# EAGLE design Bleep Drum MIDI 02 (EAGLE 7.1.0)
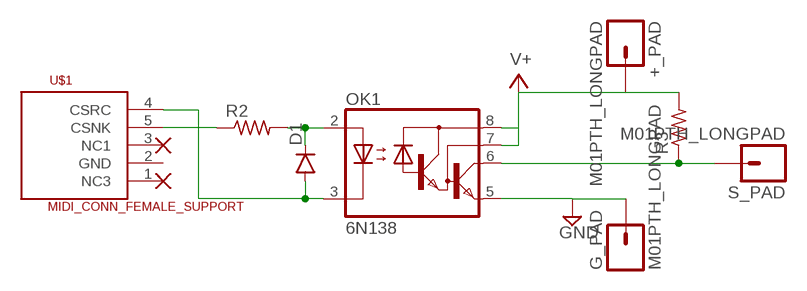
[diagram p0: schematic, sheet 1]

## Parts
+_PAD  M01PTH_LONGPAD  [1X01_LONGPAD]
D1  DIODE1N4148  [DIODE-1N4148]
G_PAD  M01PTH_LONGPAD  [1X01_LONGPAD]
OK1  6N138  [DIL08]
R2  R-US_0204/5  [0204/5]
R3  R-US_0204/5  [0204/5]
S_PAD  M01PTH_LONGPAD  [1X01_LONGPAD]
U$1  MIDI_CONN_FEMALE_SUPPORT  [DIN_5_FEMALE_SUPPORT]

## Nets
GND: G_PAD.1 OK1.5(GND)
N$1: R2.1 U$1.5(CSNK)
N$2: D1.C OK1.2(A) R2.2
N$6: OK1.6(VO) R3.1 S_PAD.1
N$8: D1.A OK1.3(C) U$1.4(CSRC)
V+: +_PAD.1 OK1.7(VB) OK1.8(VCC) R3.2
Unconnected: U$1.1(NC3) U$1.2(GND) U$1.3(NC1)

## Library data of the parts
+_PAD G_PAD S_PAD = SparkFun-Connectors:M01: Header 1
D1 = SparkFun-DiscreteSemi:DIODE: Diode
OK1 = optocoupler:6N138: MOTOROLA OPTO COUPLER; MF: VISHAY/TELEFUNKEN; MPN: 6N138; OC_FARNELL: 9860150; OC_NEWARK: 35K5294
R2 R3 = adafruit:R-US_: RESISTOR, American symbol
U$1 = SparkFun-Connectors:MIDI_CONN_FEMALE_SUPPORT: MIDI connector with strain relief (DIN-5 female)

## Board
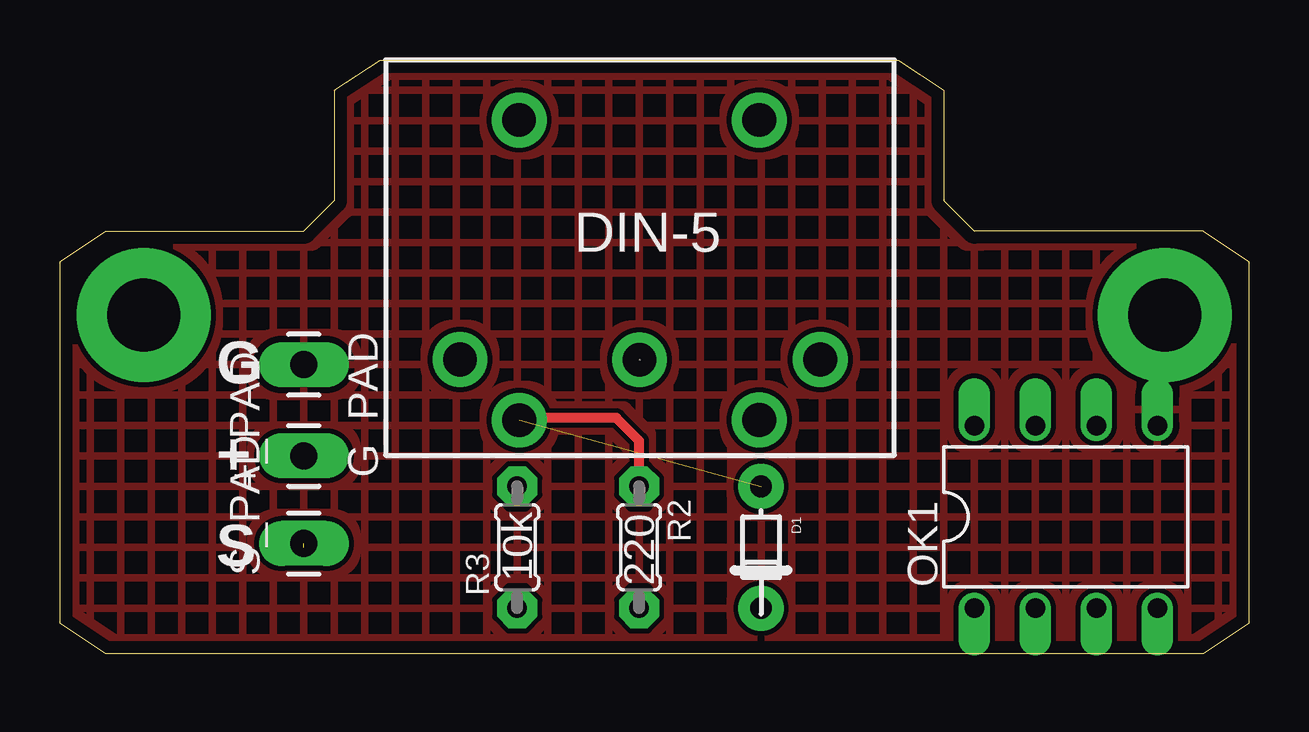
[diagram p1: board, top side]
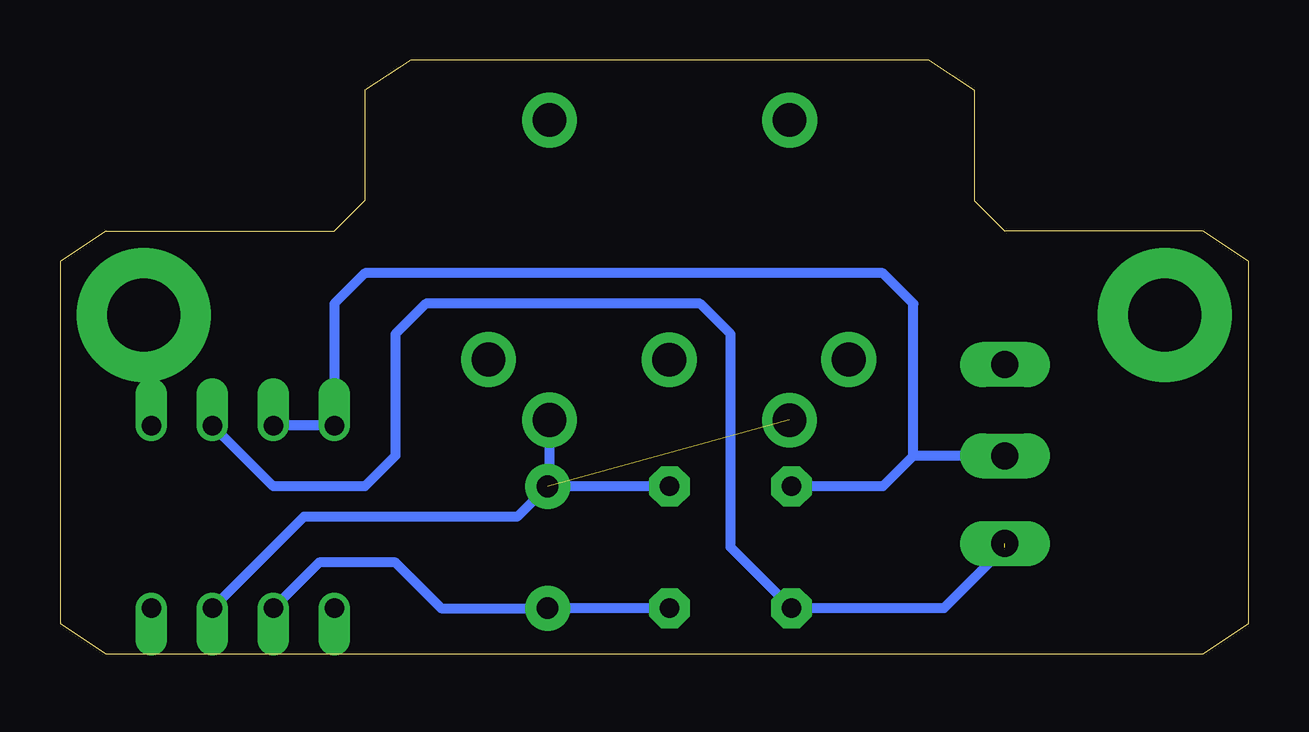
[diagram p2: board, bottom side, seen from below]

Size 49.53 x 24.77 mm. Coordinates in mm from the lower left corner, seen from the top.
Outline: 13.34,24.77 34.93,24.77 36.83,23.49 36.83,18.89 38.1,17.62 47.62,17.62 49.53,16.35 49.53,1.27 47.62,0 1.91,0 0,1.27 0,16.35 1.91,17.62 10.16,17.62 11.43,18.89 11.43,23.49 13.34,24.77
Copper layers (1*16): Top 0.035mm / dielectric 1.5mm / Bottom 0.035mm
Design rules "default": minimum track width 12mil, minimum drill 15mil, track to track 8mil, track to pad 8mil, pad to pad 8mil, via to via 8mil, smd to smd 8mil, copper to edge 20mil, drill to drill 8mil, minimum pad ring 10mil, minimum via ring 8mil, stop-mask expansion 4mil, vias tented up to drill 0mil, thermal gap 10mil

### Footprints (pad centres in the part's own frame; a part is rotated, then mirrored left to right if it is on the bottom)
1X01_LONGPAD = drill 1.118 pad 1.88 long: 1 0,0
DIODE-1N4148 = drill 0.9 pad 1.88: A -3.81,0; C 1.27,0
DIL08 = drill 0.813 offset: 1 -3.81,-3.81; 2 -1.27,-3.81; 3 1.27,-3.81; 4 3.81,-3.81; 5 3.81,3.81; 6 1.27,3.81; 7 -1.27,3.81; 8 -3.81,3.81
0204/5 = drill 0.813 pad 1.676 octagon: 1 -2.54,0; 2 2.54,0
DIN_5_FEMALE_SUPPORT = drill 1.4 pad 2.286: 1 7.94,3.6; 2 0.46,3.61; 3 -7.07,3.6; 4 5.47,6.13; 5 -4.53,6.12; 6 -4.53,-6.382; 7 5.478,-6.382

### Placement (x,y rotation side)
+_PAD  10.16,8.26 90 top
D1  29.21,3.17 270 top
G_PAD  10.16,12.07 270 top
OK1  41.91,5.71 0 top
R2  24.13,4.44 270 top
R3  19.05,4.44 90 top
S_PAD  10.16,4.6 90 top
U$1  24.61,15.88 180 top

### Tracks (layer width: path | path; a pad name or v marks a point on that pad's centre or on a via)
GND
  pour Top (hatched): -2.54,-0.64 -2.54,25.24 50.8,25.24 50.8,-1.91
N$1
  Top 0.406: R2.1 24.13,8.89 23.18,9.84 19.05,9.84
  Bottom 0.406: U$1.5 29.14,7.06 29.21,6.99 R2.1
N$2
  Bottom 0.406: OK1.2 38.73,3.81 35.56,3.81 33.66,1.91 D1.C R2.2
N$6  (1 unrouted)
  Bottom 0.406: 10.16,4.44 12.7,1.91 16.51,1.91 R3.1 | R3.1 21.59,4.44 | 21.59,4.44 R3.1 | 21.59,4.44 21.59,13.34 22.86,14.61 34.29,14.61 35.56,13.34 35.56,8.26 36.83,6.99 40.64,6.99 OK1.6
N$8  (1 unrouted)
  Bottom 0.406: OK1.3 39.37,5.71 30.48,5.71 D1.A
N$21  (via drill 3.05 pad 5.59)
  other vias: 46.04,14.13
N$89  (via drill 3.05 pad 5.59)
  other vias: 3.49,14.13
V+
  Bottom 0.406: +_PAD.1 12.7,8.26 13.97,8.26 | 13.97,8.26 13.97,14.61 15.24,15.88 36.83,15.88 38.1,14.61 OK1.8 OK1.7 | 13.97,8.26 15.24,6.99 R3.2

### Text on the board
_tsilk: G | + | S | 10k | 220

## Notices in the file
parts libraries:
SparkFun-Connectors: Licensing: CC v3.0 Share-Alike You are welcome to use this library for commercial purposes.
SparkFun-DiscreteSemi: Licensing: Creative Commons ShareAlike 4.0 International - https://creativecommons.org/licenses/by-sa/4.0
